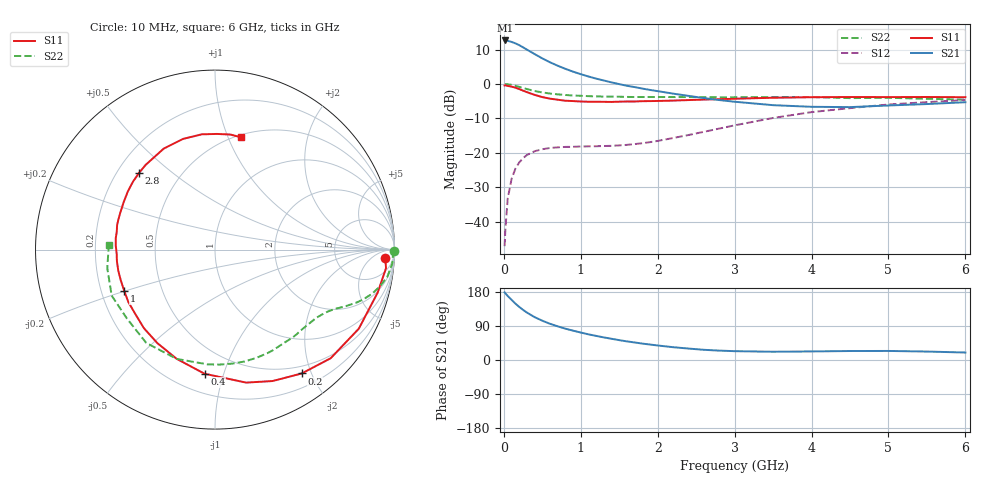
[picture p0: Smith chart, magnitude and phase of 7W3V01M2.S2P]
! Infineon Technologies  Discrete & RF Semiconductors
! BFS17W
! Si NPN RF Bipolar Junction Transistor in SOT323
! VCE = 3 V  IC = 1.2 mA
! Common Emitter S-Parameters:  August  1999
# GHz  S  MA  R  50
!  f  S11  S21  S12  S22
! GHz  MAG  ANG  MAG  ANG  MAG  ANG  MAG  ANG
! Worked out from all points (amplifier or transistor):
!   36 points, 10 MHz to 6 GHz, reference 50 ohm
!   highest |S21| = 12.6 dB at 20 MHz (marker M1)
!   |S21| within 3 dB of that: start of sweep to 325.9 MHz
!   unconditionally stable (mu >= 1): 977.4 MHz to end of sweep
!   at 250 MHz: K = 0.28, MSG = 16.1 dB, |S12| = -21.6 dB
!   at 1.4 GHz: K = 1.30, MAG = 5.9 dB, |S12| = -18.0 dB
!   at 6 GHz: K = 1.10, MAG = -2.3 dB, |S12| = -4.7 dB
!   S11 on the Smith chart (normalised r, x): 10 MHz: 20, -19; 200 MHz: 0.39, -1.86; 400 MHz: 0.32, -0.87; 1 GHz: 0.30, -0.20; 2.8 GHz: 0.29, +0.39; 6 GHz: 0.52, +1.11
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0.01  0.9498 -2.9  4.266 178.6  0.0044 88.3  0.9999 -0.4
0.02  0.9584 -6.2  4.288 175.8  0.0077 86.4  0.992 -1.8
0.05  0.9375 -14.8  4.236 169.1  0.0214 82.6  0.9904 -4.6
0.1  0.9144 -28.8  4.084 159.0  0.0416 73.4  0.9719 -9.0
0.15  0.8842 -43.2  3.893 148.9  0.0587 65.9  0.9401 -12.7
0.2  0.8425 -55.0  3.666 140.1  0.0724 60.1  0.9078 -15.8
0.25  0.7996 -66.3  3.405 132.2  0.0836 53.9  0.8733 -18.4
0.3  0.7612 -76.8  3.155 125.2  0.093 49.8  0.8438 -20.4
0.4  0.6941 -94.8  2.719 113.1  0.1054 42.9  0.7906 -23.6
0.5  0.6451 -109.3  2.354 103.7  0.1127 38.2  0.7534 -25.8
0.6  0.6119 -121.7  2.065 95.6  0.1175 35.3  0.7261 -27.9
0.7  0.5905 -132.1  1.842 88.8  0.12 33.5  0.7066 -29.9
0.8  0.5709 -141.0  1.659 82.7  0.1218 32.6  0.6918 -32.1
1  0.5561 -155.3  1.387 72.5  0.1235 32.8  0.6732 -36.1
1.1  0.5521 -162.2  1.284 67.7  0.1241 33.9  0.6657 -38.7
1.6  0.5566 173.5  0.941 49.1  0.1304 42.5  0.6485 -51.7
2.2  0.5734 152.5  0.724 33.8  0.164 56.0  0.6459 -69.0
2.8  0.6013 134.8  0.584 24.8  0.2249 62.0  0.641 -87.6
3.5  0.6311 116.9  0.492 21.8  0.3209 59.9  0.6453 -109.3
4.5  0.6464 96.5  0.461 23.7  0.4456 47.9  0.6231 -142.1
5.5  0.6468 82.4  0.511 22.3  0.5452 35.0  0.6089 -170.2
6  0.6421 77.2  0.543 19.7  0.5835 29.0  0.5924 177.4
